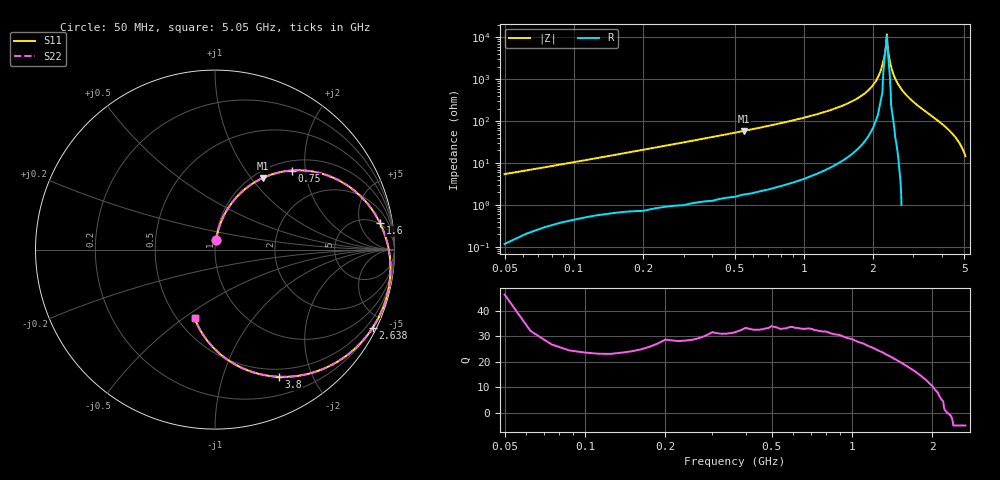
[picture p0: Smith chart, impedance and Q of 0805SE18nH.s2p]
! AVX Thin Film Operation		Date: May 2002
! Description: Accu-L® Series, Thin Film, SMD, RF Inductors
! Part Number: L0805180GEWTR
! 50 MHz  -  5.05 GHz
! Serial Measurements
# mhz S db R 50
!	S11		S21		S12		S22
!	dB	Phase	dB	Phase	dB	Phase	dB	Phase
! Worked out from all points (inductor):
!   401 points, 50 MHz to 5.05 GHz, reference 50 ohm
!   read as one part in series: L = 16.6 nH near 75 MHz
!   highest Q = 33.4 at 550 MHz (marker M1), where L = 16.9 nH
!   self-resonance near 2.275 GHz
!   S11 on the Smith chart (normalised r, x): 50 MHz: 1.01, +0.10; 750 MHz: 1.19, +1.69; 1.6 GHz: 5, +11; 2.638 GHz: 0.19, -4.26; 3.8 GHz: 0.40, -1.55; 5.05 GHz: 0.61, -0.55
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50  -25.68 84.0  -0.01 -3.2  -0.01 -3.2  -25.68 84.0
137.5  -17.47 79.1  -0.13 -8.5  -0.13 -8.5  -17.47 79.1
225  -13.37 74.2  -0.28 -13.7  -0.28 -13.7  -13.37 74.2
550  -6.35 56.2  -1.28 -31.9  -1.28 -31.9  -6.35 56.2
750  -4.23 45.8  -2.23 -42.2  -2.23 -42.2  -4.23 45.8
887.5  -3.20 39.1  -3.03 -48.8  -3.03 -48.8  -3.20 39.1
1262.5  -1.44 22.4  -5.86 -65.0  -5.86 -65.0  -1.44 22.4
1600  -0.61 9.0  -9.52 -77.7  -9.52 -77.7  -0.61 9.0
1725  -0.42 4.4  -11.33 -82.0  -11.30 -82.0  -0.42 4.4
1950  -0.20 -3.6  -15.87 -88.6  -15.90 -88.6  -0.20 -3.6
2100  -0.11 -8.8  -20.94 -91.5  -20.90 -91.5  -0.11 -8.8
2212.5  -0.08 -12.5  -28.12 -77.5  -28.10 -77.5  -0.08 -12.5
2275  -0.07 -14.6  -35.31 -17.9  -35.30 -17.9  -0.07 -14.6
2300  -0.07 -15.4  -41.60 6.0  -41.60 6.0  -0.07 -15.4
2400  -0.08 -18.7  -26.34 64.5  -26.30 64.5  -0.08 -18.7
2550  -0.13 -23.6  -18.90 65.0  -18.90 65.0  -0.13 -23.6
2637.5  -0.17 -26.4  -16.42 63.4  -16.40 63.4  -0.17 -26.4
2937.5  -0.42 -35.9  -11.20 55.7  -11.20 55.7  -0.42 -35.9
3387.5  -1.07 -50.1  -6.96 42.8  -6.96 42.8  -1.07 -50.1
3800  -2.00 -63.2  -4.55 30.7  -4.55 30.7  -2.00 -63.2
4225  -3.39 -77.1  -2.85 18.2  -2.85 18.2  -3.39 -77.1
5050  -7.99 -106.6  -0.91 -6.3  -0.91 -6.3  -7.99 -106.6
